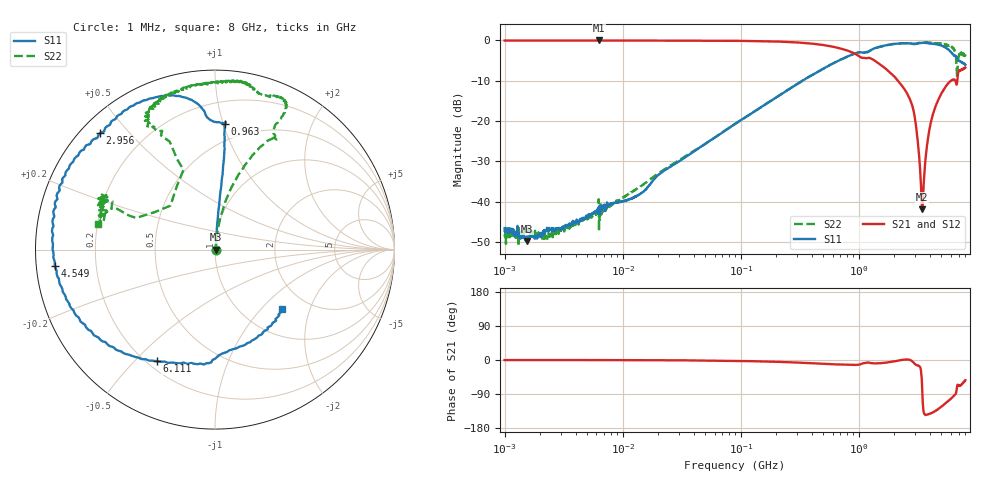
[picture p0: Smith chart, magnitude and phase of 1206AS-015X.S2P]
!s-Parameter Generated by FASTRON Sdn. Bhd.
!FASTRON P/N : 1206AS-015X
!Keysight Technologies: E5071C_MY46733604_B.14.02
!Date: Wed Nov 15 09:41:30 2023
!Version  :Rev00  Wed Nov 15 09:41:30 2023
!Data & Calibration Information:
!Freq  S11:SOLT2(ON)  S21:SOLT2(ON)  S12:SOLT2(ON)  S22:SOLT2(ON)
!PortZ  Port1:50+j0  Port2:50+j0
!When reading reference impedance value at option line is always used.
! Remarks : This data is being provided solely for informational purposes.
# Hz S dB R 50
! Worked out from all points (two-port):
!   1601 points, 1 MHz to 8 GHz, reference 50 ohm
!   highest |S21| = -0.01 dB at 6.301 MHz (marker M1); lowest = -41.9 dB at 3.447 GHz (marker M2)
!   |S21| within 3 dB of the highest: start of sweep to 884.7 MHz
!   lowest |S11| = -49.8 dB at 1.541 MHz (marker M3), VSWR 1.01, Z = 50.3 - j0.0466 ohm
!   |S11| at or under -10 dB: start of sweep to 333.4 MHz
!   |S22| runs from -51.1 to -0.4 dB; largest |S21 - S12| = 0.006
!   S11 on the Smith chart (normalised r, x): 1 MHz: 1.01, -0.00; 963 MHz: 0.37, +1.01; 2.956 GHz: 0.05, +0.42; 4.549 GHz: 0.05, -0.05; 6.111 GHz: 0.24, -0.58; 8 GHz: 1.50, -1.32
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1000000  -46.60 -17.1  -0.03 -0.2  -0.04 -0.1  -48.14 -15.6
1541011  -49.76 -8.2  -0.03 -0.2  -0.03 -0.1  -46.91 -18.3
2198553  -47.34 23.3  -0.03 -0.1  -0.04 -0.2  -48.35 41.0
4479405  -44.28 47.4  -0.04 -0.2  -0.04 -0.2  -44.95 52.2
6301378  -41.23 41.5  -0.01 -0.3  -0.05 -0.1  -47.47 42.7
1.345746e7  -38.49 77.9  -0.03 -0.4  -0.05 -0.4  -36.72 66.9
2.00676e7  -33.36 77.0  -0.04 -0.6  -0.05 -0.5  -33.01 76.3
8.994653e7  -20.66 84.5  -0.10 -2.4  -0.11 -2.3  -20.75 82.1
4.006501e8  -8.62 84.4  -0.79 -8.5  -0.80 -8.5  -8.64 74.8
9.629629e8  -3.07 85.4  -3.57 -12.9  -3.58 -12.9  -3.09 62.5
1.7949e9  -1.10 104.1  -7.66 -5.9  -7.68 -6.1  -1.10 63.5
2.530914e9  -0.71 121.9  -12.86 1.1  -12.89 0.8  -0.71 66.8
2.956409e9  -0.81 134.7  -18.47 -9.1  -18.51 -9.2  -0.92 72.4
3.446699e9  -0.58 150.2  -41.91 -80.5  -41.88 -80.6  -0.53 79.6
3.548043e9  -0.58 153.1  -35.50 -137.6  -35.52 -137.7  -0.50 80.8
3.933151e9  -0.73 164.9  -22.69 -142.2  -22.69 -142.3  -0.56 87.0
4.548578e9  -0.94 -174.3  -15.79 -132.3  -15.76 -132.5  -0.72 97.1
5.248374e9  -1.55 -149.9  -12.22 -117.7  -12.20 -117.9  -0.87 107.9
6.110812e9  -3.08 -117.7  -9.91 -100.9  -9.90 -101.2  -1.66 116.6
6.57347e9  -3.87 -97.3  -9.98 -90.8  -9.96 -91.3  -3.05 115.3
7.036128e9  -5.00 -77.4  -7.69 -68.4  -7.68 -68.9  -3.99 154.8
8e9  -6.04 -41.5  -6.78 -53.4  -6.77 -54.0  -3.48 167.7
